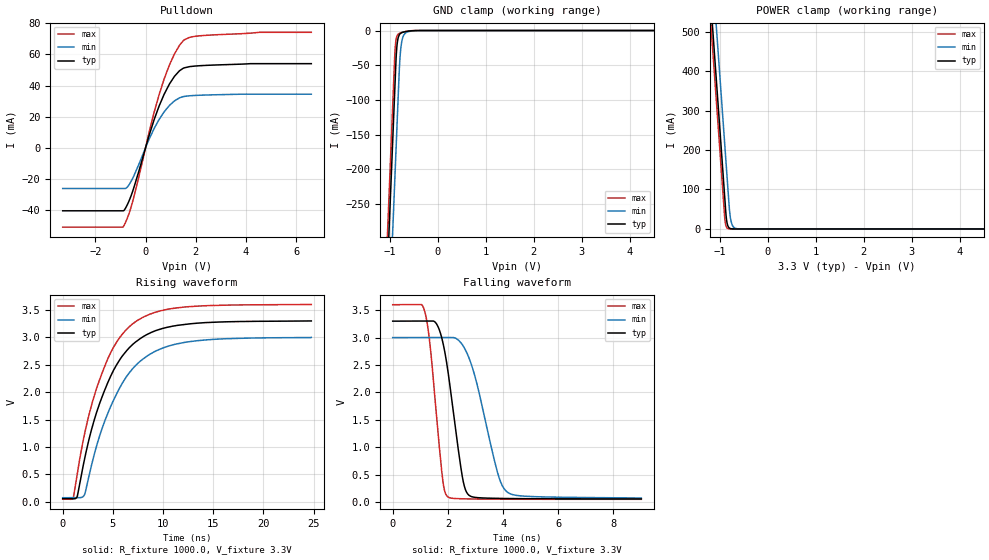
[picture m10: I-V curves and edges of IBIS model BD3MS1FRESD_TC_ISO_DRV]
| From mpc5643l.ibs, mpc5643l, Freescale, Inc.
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| *** New cell (Generated with 5.14beta1 (Sep 20 2010 13:23:23))
[Model]   BD3MS1FRESD_TC_ISO_DRV
Model_type Open_drain
Polarity   Non-Inverting
Enable   Active-Low
| CAP_THRESHOLD on pad pad is "CMOS" :
| Rising=10.0% of VDDE1   Falling=90.0% of VDDE1
| C_comp min and max val. don't necessarily correlate with the min and max pvt
| but are the smallest and greatest pad capacitance found.
| var   typ   min   max
C_comp   2.74652pF  2.56071pF  2.97794pF
Vmeas = 1.65V   | Reference voltage for timing measurements
Cref  = 50.0pF   | Timing specification test load capacitance value
Rref  = 1.0kOhm   | Timing specification test load resistance value
Vref  = 3.3V   | Timing specification test load voltage
| variable   typ   min   max
[Temperature Range] 25.0 150.0 -40.0
| variable   typ   min   max
[Voltage Range] 3.3V 3.0V 3.6V
| variable   typ   min   max
[POWER Clamp Reference] 3.3V 3.0V 3.6V
| variable   typ   min   max
[GND Clamp Reference] 0V 0V 0V
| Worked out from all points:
|   slope of the pulldown table from 0 to 0.495 V, typ, clamps not added: 19.9 ohm
|   GND clamp passes 1 mA (typ) near -0.63 V on its own axis
|   POWER clamp passes 1 mA (typ) near -0.78 V on its own axis
|   rising waveform, R_fixture 1000.0, V_fixture 3.3V: 20-80 % time 3.82ns typ, 4.04ns min, 3.61ns max; typ from 0.056 V to 3.3 V
|   falling waveform, R_fixture 1000.0, V_fixture 3.3V: 20-80 % time 529ps typ, 824ps min, 388ps max; typ from 3.3 V to 0.056 V
[POWER Clamp]
-3.3V     4.162A     4.297A     4.11A
-1.21V    609.4mA    743.8mA    556.6mA
-1.14V    490.4mA    624.8mA    437.6mA
-1.07V    371.4mA    505.8mA    318.6mA
-900mV    82.42mA    216.8mA    29.59mA
-870mV    32.81mA    165.8mA    6.648mA
-830mV    6.917mA    97.75mA    908uA
-800mV    2.152mA    48.46mA    204uA
-760mV    453.6uA    16.18mA    27.89uA
-710mV    64.8uA     4.107mA    2.322uA
-630mV    2.882uA    457.8uA    44.65nA
6.6V      0A         0A         0A
[GND Clamp]
-3.3V     -4.17A     -4.3A      -4.118A
-1.08V    -395.6mA   -526mA     -344.2mA
-900mV    -89.61mA   -220mA     -38.24mA
-880mV    -55.61mA   -186mA     -17.63mA
-860mV    -27.99mA   -152mA     -9.68mA
-830mV    -11.42mA   -101mA     -5.557mA
-800mV    -5.861mA   -51.79mA   -4.091mA
-790mV    -4.948mA   -40.18mA   -3.778mA
-760mV    -3.359mA   -19.29mA   -3.024mA
-710mV    -2.143mA   -6.577mA   -2.024mA
-490mV    -149.6uA   -443.8uA   -71.63uA
6.6V      87.85pA    30.93nA    1.364pA
| variable   typ   min   max
[Pullup Reference] 3.3V 3.0V 3.6V
| variable   typ   min   max
[Pulldown Reference] 0V 0V 0V
[Pullup]
-3.3V     0A         0A         0A
0V        0A         0A         0A
6.6V      0A         0A         0A
[Pulldown]
-3.3V     -40.62mA   -26.25mA   -51.14mA
-890mV    -40.62mA   -26.25mA   -50.91mA
-740mV    -37.11mA   -25.58mA   -45.87mA
-540mV    -29.27mA   -20.52mA   -36.12mA
340mV     17.99mA    12.32mA    22.74mA
740mV     34.39mA    23.07mA    44.22mA
1.15V     45.9mA     30.1mA     60.29mA
1.35V     49.48mA    32.06mA    65.84mA
1.55V     51.41mA    33.01mA    69.46mA
1.96V     52.51mA    33.6mA     71.63mA
2.57V     53.06mA    33.95mA    72.44mA
6.6V      54.05mA    34.41mA    74.22mA
[Ramp]
dV/dt_r 1.94601V/3.81532ns 1.75552V/4.04374ns 2.13032V/3.61453ns
dV/dt_f 1.94616V/528.62377ps 1.75575V/824.39258ps 2.13043V/388.41846ps
R_load = 1000.0
| Removed startup time: 0s 0s 0s  .
| Removed end time: 24.77ns.
[Rising Waveform]
R_fixture   = 1000.0
V_fixture   = 3.3V
V_fixture_min = 3.0V
V_fixture_max = 3.6V
0s        56.39mV    73.72mV    49.27mV
1.055ns   53.03mV    73.67mV    75.36mV
1.46ns    105.4mV    72.29mV    526.8mV
2.155ns   760.7mV    122.8mV    1.218V
3.175ns   1.512V     885.7mV    1.953V
4.525ns   2.188V     1.629V     2.622V
7.085ns   2.889V     2.451V     3.263V
9.155ns   3.115V     2.74V      3.453V
11.93ns   3.231V     2.902V     3.55V
24.78ns   3.3V       3V         3.6V
| Removed startup time: 0s 0s 0s  .
| Removed end time: 9.0ns.
[Falling Waveform]
R_fixture   = 1000.0
V_fixture   = 3.3V
V_fixture_min = 3.0V
V_fixture_max = 3.6V
0s        3.3V       3V         3.6V
1.155ns   3.302V     3.001V     3.488V
1.365ns   3.303V     3.001V     2.814V
1.8ns     2.95V      3.002V     455.1mV
1.995ns   2.41V      3.002V     95.04mV
2.525ns   456.7mV    2.869V     58.89mV
2.79ns    114.2mV    2.596V     56.17mV
3.785ns   66.63mV    562.7mV    51.79mV
4.135ns   63.93mV    188.8mV    51.1mV
9.01ns    56.39mV    73.72mV    49.27mV
